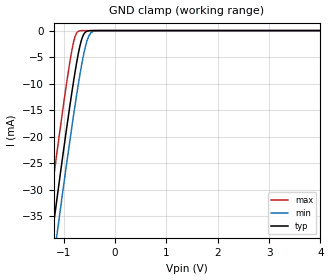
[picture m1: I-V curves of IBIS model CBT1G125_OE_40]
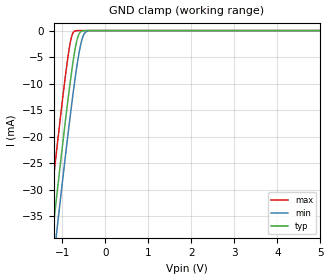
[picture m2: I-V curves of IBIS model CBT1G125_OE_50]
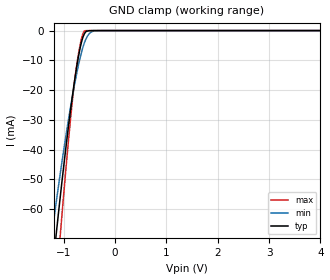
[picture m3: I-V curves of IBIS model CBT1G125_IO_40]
| TEXAS INSTRUMENTS INCORPORATED
| Standard Linear and Logic Group
| IBIS Model of SN74CBT1G125
| SINGLE FET BUS SWITCH
| This file contains package information for the following:
|  SOT 5-pin (DBV) package as [Component] CBT1G125_DBV
|  SOT 5-pin (DCK) package as [Component] CBT1G125_DCK
| This device can be powered at the following Vccs:
|  4 volt Vcc
|  5 volt Vcc
| This file provides unique models under the [Model Selector] for each Vcc.
| For operation at a specific Vcc, select the appropriate model after each
| [Model Selector] keyword.
[IBIS Ver]   3.2
[Comment char]  |_char
[File Name]   sn74cbt1g125.ibs
[File Rev]   1.1 | x_die
[Date]   January 30, 2004
[Source]   Data created from TI-SPICE simulations at TI-SLL.
[Notes]   The following is an IBIS list for the CBT1G125.
   Please contact sllibis@ti.com with questions and
   comments concerning SLL IBIS models.
   - FILE REV HISTORY
   - 1.1 Release IBIS file on 02/03/04
   - Power clamp data deleted as there is no power-clamp diode.
   - Non-monotonic data due to FET characteristics.
[Disclaimer] Property of Texas Instruments Incorporated.  Unauthorized
   reproduction and/or distribution is strictly prohibited.
   This product is protected under copyright law.
   Created  2004, (C) Copyright  2004, Texas Instruments
   Incorporated, All Rights Reserved
   UNLESS THERE IS A SIGNED, WRITTEN AGREEMENT TO THE
   CONTRARY, TEXAS INSTRUMENTS (TI) IS PROVIDING THE IBIS
   MODELS  AND WITHOUT ANY WARRANTY, EXPRESSED OR
   IMPLIED.  TI assumes no liability for:
   1) the accuracy of the IBIS models provided to your
   company;
   2) the proper functioning of these IBIS Models in your
   design or for any resulting applications; or
   3) infringement of patents, copyrights or intellectual
   property rights resulting from your use of these IBIS
   models.
   TI provides IBIS Models as a service to our customers.
   You and your company shall not distribute, sell or give
   these models to anyone else without prior written
   permission from TI.
   TI reserves the right to make changes to our products or
   to discontinue any semiconductor product or service
   without notice, and advises our customers to obtain the
   latest version of relevant information to verify, before
   placing orders, that the information being relied on is
   current.
   Please be aware that your receipt and use of the IBIS
   information provided shall serve as acceptance of these
   terms and conditions.  If you do not accept these terms,
   you should return or destroy the IBIS models and any
   other accompanying information immediately.
| Component CBT1G125_DBV 5-pin SOT
[Component]   CBT1G125_DBV
[Manufacturer]   Texas Instruments, Inc.
[Package]
|   typ   min   max
R_pkg   2.500e-02   2.100e-02   2.900e-02
L_pkg   1.529e-09   1.312e-09   1.906e-09
C_pkg   1.560e-13   1.100e-13   2.400e-13
[Pin]   signal_name   model_name   R_pin   L_pin   C_pin
1   NOE   CBT1G125_OE   2.100e-02   1.511e-09   1.440e-13
2   A   CBT1G125_IO   2.300e-02   1.312e-09   1.380e-13
3   GND   GND   2.900e-02   1.906e-09   2.400e-13
4   B   CBT1G125_IO   2.600e-02   1.541e-09   1.500e-13
5   VCC   POWER   2.500e-02   1.374e-09   1.100e-13
| Component CBT1G125_DCK 5-pin SOT
[Component]   CBT1G125_DCK
[Manufacturer]   Texas Instruments, Inc.
[Package]
|   typ   min   max
R_pkg   2.000e-02   1.700e-02   2.500e-02
L_pkg   9.980e-10   8.810e-10   1.069e-09
C_pkg   1.460e-13   1.180e-13   2.050e-13
[Pin]   signal_name   model_name   R_pin   L_pin   C_pin
1   NOE   CBT1G125_OE   1.900e-02   1.069e-09   1.620e-13
2   A   CBT1G125_IO   1.800e-02   8.810e-10   1.210e-13
3   GND   GND   1.700e-02   1.031e-09   2.050e-13
4   B   CBT1G125_IO   2.000e-02   9.600e-10   1.240e-13
5   VCC   POWER   2.500e-02   1.049e-09   1.180e-13
[Series Switch Groups]
| Function Group States
On  1 /   | A->B NOE LOW
Off 1 /   | NOE HIGH
[Series Pin Mapping]   pin_2   model_name   function_table_group
2   4   CBT1G125_IO_40_S   1
| 2   4   CBT1G125_IO_50_S   1
| Model CBT1G125_OE
[Model Selector]   CBT1G125_OE
CBT1G125_OE_40   4 volt Vcc
CBT1G125_OE_50   5 volt Vcc
| Model CBT1G125_IO
[Model Selector]   CBT1G125_IO
CBT1G125_IO_40   4 volt Vcc
CBT1G125_IO_50   5 volt Vcc
| Model CBT1G125_IO_S
[Model Selector]   CBT1G125_IO_S
CBT1G125_IO_40_S   4 volt Vcc_S
CBT1G125_IO_50_S   5 volt Vcc_S
[Model]   CBT1G125_IO_40_S
Model_type  Series_switch
| variable   typ   min   max
C_comp   0   0   0
[Temperature Range]   40   100   -40
| Ambient temperature   25   85   -40
[Voltage range]   4   4   4
[On]
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[Off]
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[Model]   CBT1G125_IO_50_S
Model_type  Series_switch
| variable   typ   min   max
C_comp   0   0   0
[Temperature Range]   40   100   -40
| Ambient temperature   25   85   -40
[Voltage range]   5   4.5   5.5
[On]
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[Off]
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| Models and submodels in the file (6): CBT1G125_OE_40 (Input), CBT1G125_OE_50 (Input), CBT1G125_IO_40_S (Series_switch), CBT1G125_IO_40 (Terminator), CBT1G125_IO_50_S (Series_switch), CBT1G125_IO_50 (Terminator)
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[Model]   CBT1G125_OE_40
Model_type  Input
Vinl = 0.8
Vinh = 2
| variable   typ   min   max
C_comp   1.06pF   0.89pF   1.20pF
[Temperature Range]   40   100   -40
| Ambient temperature   25   85   -40
[Voltage range]   4   4   4
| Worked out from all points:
|   GND clamp passes 1 mA (typ) near -0.63 V on its own axis
[GND Clamp]
| CBT1G125_OE_40
|   Voltage   I(typ)   I(min)   I(max)
-4V       -250mA     -256.3mA   -242mA
-1.365V   -48.74mA   -55.5mA    -40.02mA
-1.31V    -44.67mA   -51.45mA   -35.94mA
-1.21V    -37.33mA   -44.12mA   -28.58mA
-1.125V   -31.16mA   -37.95mA   -22.41mA
-850mV    -12.12mA   -18.65mA   -4.156mA
-780mV    -7.787mA   -14.05mA   -1.143mA
-710mV    -4.013mA   -9.713mA   -111.7uA
-630mV    -1.091mA   -5.305mA   -4.37uA
-555mV    -159.3uA   -2.168mA   -194.1nA
-405mV    -1.677uA   -91.86uA   -391.1pA
4V        28.91pA    2.706nA    22.55pA
[Model]   CBT1G125_OE_50
Model_type  Input
Vinl = 0.8
Vinh = 2
| variable   typ   min   max
C_comp   1.22pF   0.87pF   3.53pF
[Temperature Range]   40   100   -40
| Ambient temperature   25   85   -40
[Voltage range]   5   4.5   5.5
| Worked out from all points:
|   GND clamp passes 1 mA (typ) near -0.63 V on its own axis
[GND Clamp]
| CBT1G125_OE_50
|   Voltage   I(typ)   I(min)   I(max)
-5V       -327.3mA   -333.4mA   -319.5mA
-1.365V   -48.74mA   -55.5mA    -40.02mA
-1.325V   -45.78mA   -52.55mA   -37.05mA
-1.215V   -37.7mA    -44.48mA   -28.94mA
-1.125V   -31.16mA   -37.95mA   -22.41mA
-850mV    -12.12mA   -18.65mA   -4.156mA
-780mV    -7.787mA   -14.05mA   -1.143mA
-710mV    -4.013mA   -9.713mA   -111.7uA
-625mV    -978.1uA   -5.059mA   -3.551uA
-540mV    -103.1uA   -1.713mA   -104.2nA
-380mV    -774.4nA   -49uA      -140.7pA
5V        35.05pA    2.725nA    24.17pA
[Model]   CBT1G125_IO_40
Model_type  Terminator
| variable   typ   min   max
C_comp   3.38pF   2.88pF   4.03pF
| C_tri-state   3.38pF   2.88pF   4.03pF
[Temperature Range]   40   100   -40
| Ambient temperature   25   85   -40
[Voltage range]   4   4   4
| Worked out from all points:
|   GND clamp passes 1 mA (typ) near -0.60 V on its own axis
[GND Clamp]
| CBT1G125_IO_40
|   Voltage   I(typ)   I(min)   I(max)
-4V       -635.5mA   -514.1mA   -806.6mA
-1.25V    -85.31mA   -70.73mA   -108mA
-1.215V   -79.45mA   -66.2mA    -100.2mA
-1.145V   -67.96mA   -57.35mA   -84.91mA
-1.075V   -56.82mA   -48.79mA   -70.04mA
-1.045V   -52.17mA   -45.22mA   -63.81mA
-885mV    -28.93mA   -27.43mA   -32.63mA
-780mV    -15.69mA   -17.2mA    -15.64mA
-680mV    -5.731mA   -9.023mA   -4.668mA
-595mV    -970.9uA   -3.956mA   -98.27uA
-335mV    -289.1nA   -21.08uA   -2.087nA
4V        41.49pA    2.944nA    19.54pA
